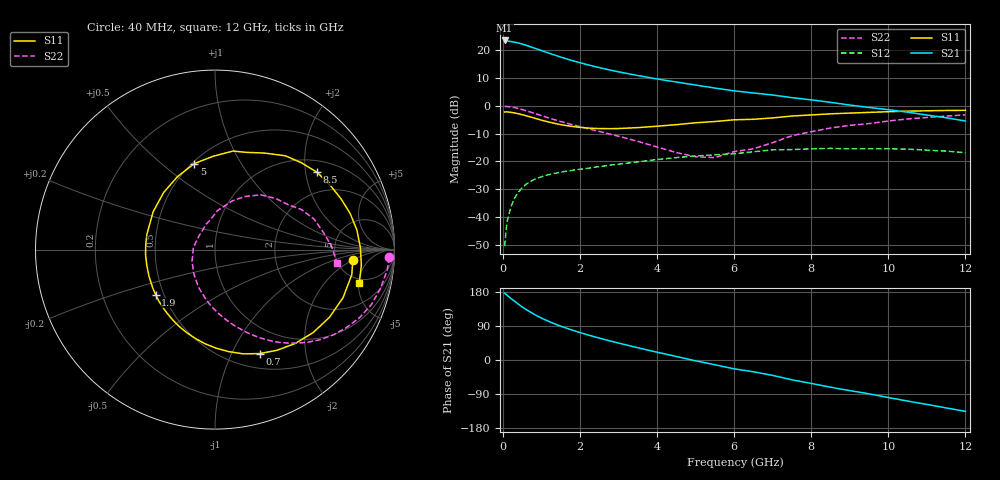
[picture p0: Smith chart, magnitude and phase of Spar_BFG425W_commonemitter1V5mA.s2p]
! Filename: 15bfg425.001
! BFG425W Field C1
! V1=8.342E-001V,V2=1.000E+000V, I1=7.034E-005A, I2=5.000E-003A
# GHz  S  MA  R 50
!  S11  S21  S12  S22
!Freq(GHz)  Mag  Ang  Mag  Ang  Mag  Ang  Mag  Ang
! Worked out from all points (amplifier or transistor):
!   44 points, 40 MHz to 12 GHz, reference 50 ohm
!   highest |S21| = 23.4 dB at 40 MHz (marker M1)
!   |S21| within 3 dB of that: start of sweep to 868.5 MHz
!   unconditionally stable (mu >= 1): 2.398 GHz to end of sweep
!   at 700 MHz: K = 0.34, MSG = 24.3 dB, |S12| = -27.3 dB
!   at 2.4 GHz: K = 1.00, MAG = 17.9 dB, |S12| = -22.0 dB
!   at 12 GHz: K = 1.49, MAG = 1.5 dB, |S12| = -16.9 dB
!   S11 on the Smith chart (normalised r, x): 40 MHz: 7.13, -1.98; 700 MHz: 0.67, -1.29; 1.9 GHz: 0.45, -0.27; 5 GHz: 0.51, +0.65; 8.5 GHz: 1.32, +2.32; 12 GHz: 4.37, -5.09
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0.04  0.77 -4.2  14.84 176.1  0.003 74.8  0.971 -2.5
0.1  0.775 -10.4  14.54 171.2  0.008 84.9  0.967 -6.5
0.2  0.762 -20.6  14.21 162.7  0.015 77.8  0.947 -13.3
0.3  0.741 -30.6  13.84 154.9  0.022 72.3  0.923 -19.5
0.4  0.716 -40.2  13.34 147.1  0.028 67.0  0.889 -25.4
0.5  0.688 -49.5  12.79 139.8  0.034 62.1  0.851 -30.7
0.6  0.659 -58.3  12.14 133.2  0.039 57.8  0.813 -35.7
0.7  0.631 -66.7  11.5 127.0  0.043 53.7  0.773 -40.4
0.9  0.574 -82.2  10.33 115.6  0.05 47.3  0.697 -48.4
1.2  0.506 -102.8  8.727 101.3  0.058 40.0  0.599 -58.2
1.5  0.457 -121.1  7.456 89.2  0.064 34.9  0.519 -66.3
1.9  0.415 -142.8  6.164 75.4  0.071 29.9  0.437 -75.6
2.2  0.397 -157.7  5.425 66.3  0.075 26.8  0.387 -82.2
2.6  0.388 -176.0  4.653 55.1  0.082 23.1  0.331 -91.0
3  0.389 167.4  4.054 44.6  0.089 19.4  0.282 -100.3
3.5  0.404 148.6  3.476 32.3  0.098 14.4  0.229 -113.6
4.5  0.457 117.3  2.657 9.2  0.117 2.7  0.144 -152.7
5  0.493 103.6  2.348 -2.2  0.125 -4.5  0.121 174.1
6.5  0.57 71.8  1.691 -31.1  0.149 -20.4  0.168 98.8
8.5  0.714 37.1  1.149 -71.8  0.171 -54.8  0.398 50.0
10.5  0.798 7.8  0.765 -108.4  0.166 -88.0  0.578 17.1
12  0.825 -13.0  0.532 -135.5  0.143 -116.8  0.685 -6.4
